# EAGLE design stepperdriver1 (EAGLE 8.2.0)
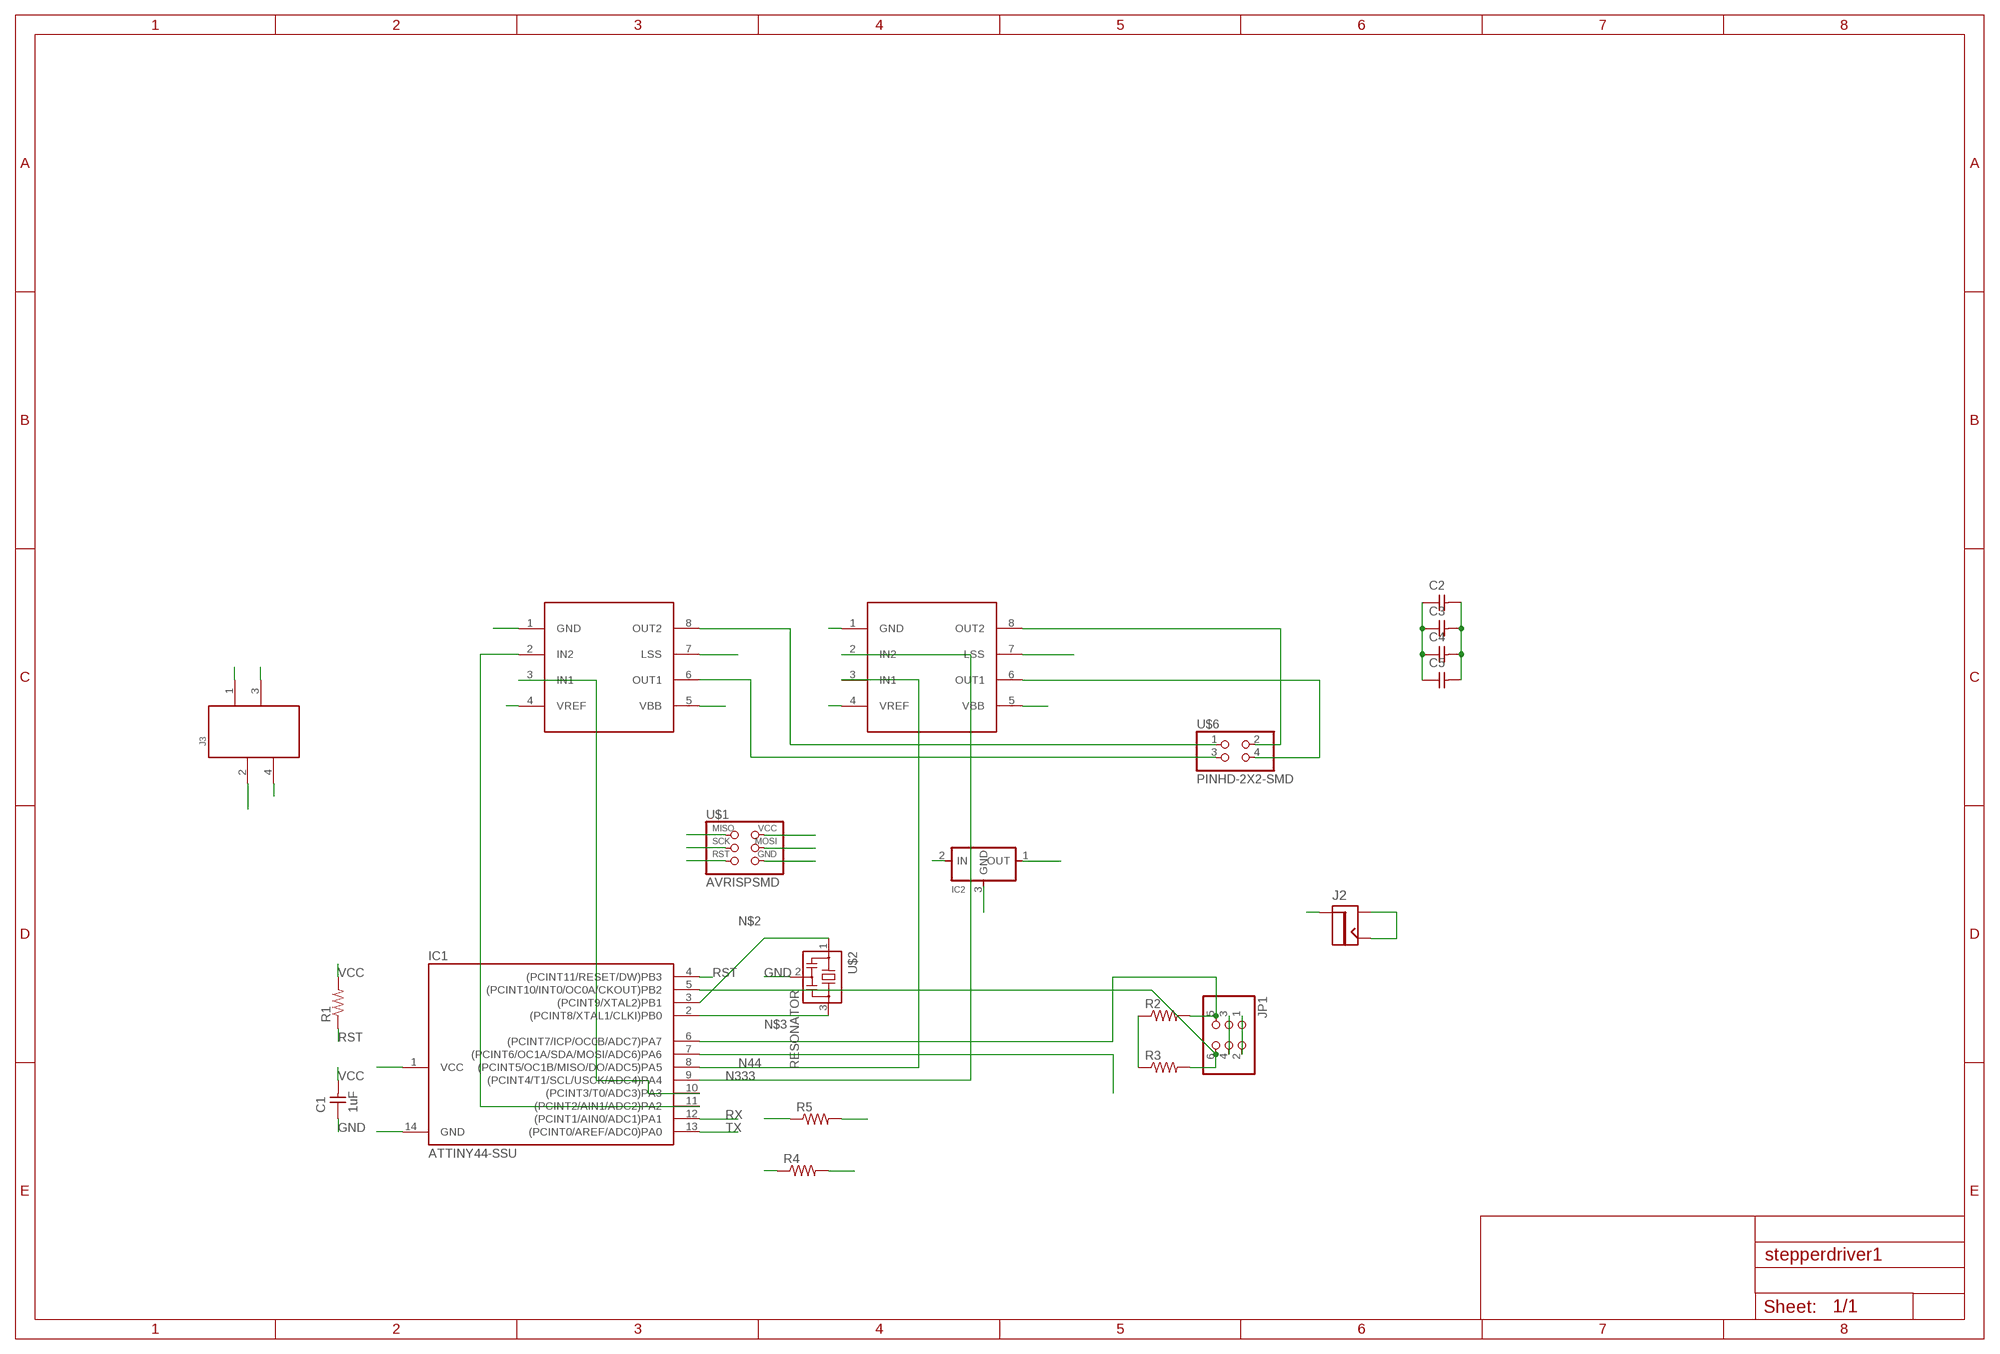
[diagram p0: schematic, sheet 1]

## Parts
C1  1uF  CAP-UNPOLARIZEDFAB  [C1206FAB]
C2  CAP-UNPOLARIZEDFAB  [C1206FAB]
C3  CAP-UNPOLARIZEDFAB  [C1206FAB]
C4  CAP-UNPOLARIZEDFAB  [C1206FAB]
C5  CAP-UNPOLARIZEDFAB  [C1206FAB]
IC1  ATTINY44-SSU  [SOIC14]
IC2  REGULATORSOT23  [SOT23]
J2  JACK2.1MM  [JACK_2.1MM]
J3  61000418321  [61000418321]
JP1  PINHD-2X3-SMD  [2X03SMD]
R1  RES-US1206FAB  [R1206FAB]
R2  RES-US1206FAB  [R1206FAB]
R3  RES-US1206FAB  [R1206FAB]
R4  RES-US1206FAB  [R1206FAB]
R5  RES-US1206FAB  [R1206FAB]
U$1  AVRISPSMD  [2X03SMD]
U$2  RESONATOR  [EFOBM]
U$4  A4953-H-BRIDGE-MOTOR-DRIVER  [SOIC8]
U$5  A4953-H-BRIDGE-MOTOR-DRIVER  [SOIC8]
U$6  PINHD-2X2-SMD  [2X02SMD]

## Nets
GND: C1.1 C2.1 C3.1 C4.1 C5.1 IC1.14(GND) IC2.3(GND) J2.CONTACT J2.SHUNT J3.2 JP1.1 JP1.2 R2.1 R3.1 R4.1 R4.2 R5.1 R5.2 U$1.6(GND) U$2.2 U$4.1(GND) U$4.7(LSS) U$5.1(GND) U$5.7(LSS)
MISO: IC1.8((PCINT5/OC1B/MISO/DO/ADC5)PA5) U$1.1(MISO) U$5.3(IN1)
MOSI: IC1.7((PCINT6/OC1A/SDA/MOSI/ADC6)PA6) U$1.4(MOSI)
N44: IC1.6((PCINT7/ICP/OC0B/ADC7)PA7) JP1.5 R2.2
N333: IC1.5((PCINT10/INT0/OC0A/CKOUT)PB2) JP1.6 R3.2
N$1: U$5.6(OUT1) U$6.4
N$2: IC1.3((PCINT9/XTAL2)PB1) U$2.1
N$3: IC1.2((PCINT8/XTAL1/CLKI)PB0) U$2.3
N$4: U$5.8(OUT2) U$6.2
N$5: U$4.8(OUT2) U$6.1
N$6: U$4.6(OUT1) U$6.3
N$9: IC1.10((PCINT3/T0/ADC3)PA3) U$4.3(IN1)
N$10: IC1.11((PCINT2/AIN1/ADC2)PA2) U$4.2(IN2)
RST: IC1.4((PCINT11/RESET/DW)PB3) R1.1 U$1.5(RST)
RX: IC1.12((PCINT1/AIN0/ADC1)PA1) J3.3
SCK: IC1.9((PCINT4/T1/SCL/USCK/ADC4)PA4) U$1.3(SCK) U$5.2(IN2)
TX: IC1.13((PCINT0/AREF/ADC0)PA0) J3.4
VBB: C2.2 C3.2 C4.2 C5.2 IC2.2(IN) J2.PIN U$4.5(VBB) U$5.5(VBB)
VCC: C1.2 IC1.1(VCC) IC2.1(OUT) J3.1 JP1.3 JP1.4 R1.2 U$1.2(VCC) U$4.4(VREF) U$5.4(VREF)

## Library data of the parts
C1-C5 = fab:CAP-UNPOLARIZED
IC1 = fab:ATTINY44
IC2 = fab:REGULATOR
J2 = fab:JACK
J3 = EAGLE-BOARD-TO-BOARD_CONNECTORS-rev16c:61000418321: WR-PHD 2.54mm SMT Pin Header, 4 Pins =>Code : Con_BTB_PHD_2.54_1_SMT_61000418321 Details see: http://katalog.we-online.de/en/em/610_0xx_182_21 Created 2014-05-29, Karrer Zheng 2014 (C) Würth Elektronik
JP1 = fab:PINHD-2X3-SMD: PIN HEADER
R1-R5 = fab:RES-US: Resistor (US Symbol)
U$1 = fab:AVRISP
U$2 = fab:RESONATOR
U$4 U$5 = fab:A4953-H-BRIDGE-MOTOR-DRIVER
U$6 = fab:PINHD-2X2-SMD

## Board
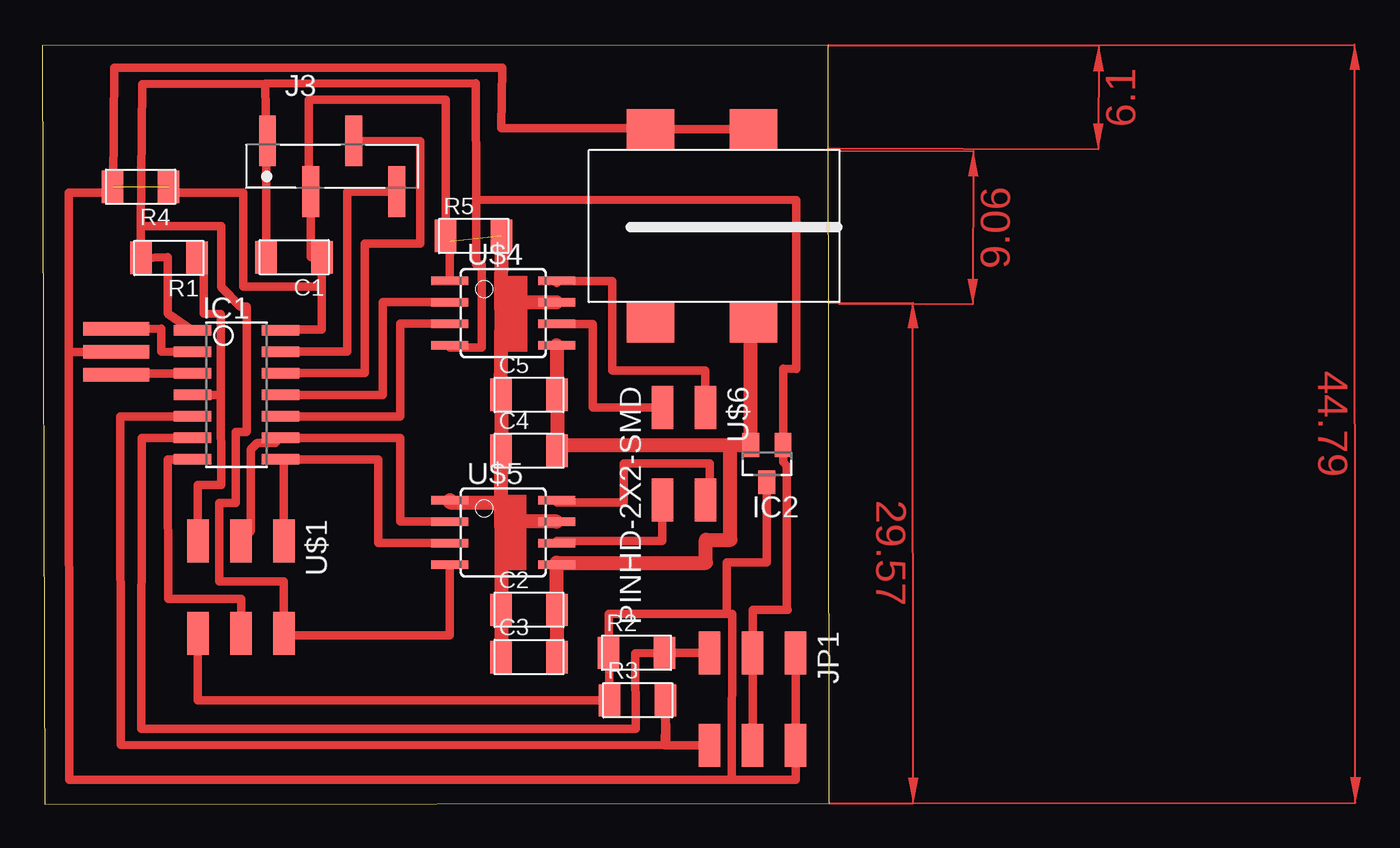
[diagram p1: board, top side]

Size 46.47 x 44.87 mm. Coordinates in mm from the lower left corner, seen from the top.
Outline: 0.14,0 46.47,0.08 46.42,44.87 0,44.84 0.14,0
Copper layers (1*16): Top 0.035mm / dielectric 1.5mm / Bottom 0.035mm
Design rules "default *": minimum track width 10mil, minimum drill 24mil, track to track 16mil, track to pad 16mil, pad to pad 16mil, via to via 16mil, smd to smd 16mil, copper to edge 40mil, drill to drill 8mil, minimum pad ring 10mil, minimum via ring 8mil, stop-mask expansion 4mil, vias tented up to drill 0mil, thermal gap 10mil

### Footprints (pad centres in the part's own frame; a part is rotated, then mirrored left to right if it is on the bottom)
C1206FAB = smd 1.27 x 1.905: 1 -1.651,0; 2 1.651,0
SOIC14 = smd 0.61 x 2.21: 1 -3.81,-2.603; 2 -2.54,-2.603; 3 -1.27,-2.603; 4 0,-2.603; 5 1.27,-2.603; 6 2.54,-2.603; 7 3.81,-2.603; 8 3.81,2.603; 9 2.54,2.603; 10 1.27,2.603; 11 0,2.603; 12 -1.27,2.603; 13 -2.54,2.603; 14 -3.81,2.603
SOT23 = smd 1 x 1.4: 1 -0.95,-1.1; 2 0.95,-1.1; 3 0,1.1
JACK_2.1MM = smd 2.388 x 2.794: CONTACT 5.766,-2.413; PIN -5.639,-2.413; PIN1 -5.639,3.683; SHUNT 5.766,3.683
61000418321 = smd 1 x 3: 1 -3.81,1.5; 2 -1.27,-1.5; 3 1.27,1.5; 4 3.81,-1.5
2X03SMD = smd 2.54 x 1.27: 1 -2.54,2.54; 2 2.92,2.54; 3 -2.54,0; 4 2.92,0; 5 -2.54,-2.54; 6 2.92,-2.54
R1206FAB = smd 1.27 x 1.905: 1 -1.651,0; 2 1.651,0
EFOBM = smd 0.8 x 3.9: 1 -1.35,0; 2 0,0; 3 1.35,0
SOIC8 = smd 0.5 x 2.2: 1 -1.905,-3.154; 2 -0.645,-3.154; 3 0.625,-3.154; 4 1.895,-3.154; 5 1.905,3.154; 6 0.635,3.154; 7 -0.635,3.154; 8 -1.905,3.154
2X02SMD = smd 2.54 x 1.27: 1 -2.54,1.27; 2 2.92,1.27; 3 -2.54,-1.27; 4 2.92,-1.27

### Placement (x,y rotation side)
C1  14.87,32.33 180 top
C2  28.74,11.51 0 top
C3  28.74,8.71 0 top
C4  28.74,20.9 0 top
C5  28.74,24.21 0 top
IC1  11.47,24.21 270 top
IC2  42.79,20.14 180 top
J2  39.59,34.12 90 top
J3  17.11,37.71 0 top
JP1  41.95,6.43 270 top
R1  7.47,32.3 180 top
R2  35.09,8.97 0 top
R3  35.15,6.16 0 top
R4  5.8,36.5 180 top
R5  25.47,33.59 0 top
U$1  11.72,13.03 270 top
U$2  4.36,26.75 90 top
U$4  27.22,29.03 270 top
U$5  27.22,16.08 270 top
U$6  37.88,20.9 270 top

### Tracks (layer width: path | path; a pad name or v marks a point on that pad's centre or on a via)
GND  (2 unrouted)
  Top 0.508: JP1.1 JP1.2 44.49,1.46 40.7,1.46 | IC2.3 42.79,14.3 40.42,14.3 40.42,11.25 | 40.42,11.25 33.44,11.25 R2.1 R3.1 9.17,6.15 U$1.6 | U$2.2 1.56,26.75 | 1.56,26.75 1.59,1.46 40.7,1.46 | 40.42,11.25 40.74,11.25 40.7,1.46 | 1.56,26.75 1.56,36.14 4.15,36.14 R4.2 4.18,36.5 4.24,43.52 27.17,43.52 27.1,39.95 35.9,39.95 J2.SHUNT J2.CONTACT | IC1.14 14.07,28.07 16.51,28.07 16.51,30.61 | 16.51,30.61 16.51,32.33 C1.1 15.84,32.33 J3.2 15.74,36.21 15.74,41.66 23.82,41.66 R5.1 24.06,33.25 U$4.1 | R4.1 7.46,36.14 11.85,36.14 11.85,30.61 16.51,30.61
  Top 0.813: 27.09,17.86 C4.1 C5.1 27.04,24.21 27.09,29.34 | 27.09,16.47 27.09,17.86 | 27.09,16.47 C2.1 C3.1 | U$5.1 24.06,17.86 27.09,17.86 | 27.09,29.34 R5.2 | U$4.7 27.41,29.67 27.09,29.34 | U$5.7 27.33,16.71 27.09,16.47
MISO
  Top 0.508: U$5.3 19.85,15.45 19.85,20.4 IC1.8 14.26,20.4 U$1.1
MOSI
  Top 0.508: IC1.7 7.4,20.4 7.44,12.15 11.76,12.15 U$1.4
N44
  Top 0.508: JP1.5 R2.2 35,8.93 35.03,4.47 5.86,4.47 5.88,21.67 IC1.6
N333
  Top 0.508: JP1.6 36.74,3.51 R3.2 36.84,3.51 4.62,3.52 4.61,22.94 IC1.5
N$1
  Top 0.508: U$5.6 30.37,15.57 36.61,15.57 U$6.4
N$2
  Top 0.508: U$2.1 3.85,25.48 IC1.3
N$3
  Top 0.508: IC1.2 7.02,26.77 7.02,28.12 U$2.3
N$4
  Top 0.508: U$5.8 30.37,17.86 34.33,17.86 34.33,20.14 39.41,20.14 39.41,17.6 39.15,17.6 U$6.2
N$5
  Top 0.508: 30.37,30.81 U$4.8 33.66,30.94 33.66,25.63 39.15,25.63 U$6.1
N$6
  Top 0.508: U$4.6 32.51,28.4 32.51,23.46 36.61,23.46 U$6.3
N$9
  Top 0.508: IC1.10 21.12,22.94 21.12,28.41 U$4.3
N$10
  Top 0.508: IC1.11 20.1,24.21 20.1,29.68 U$4.2
RST
  Top 0.508: U$1.5 9.18,18.87 10.55,18.87 10.53,24.2 | 10.53,24.2 IC1.4 | 10.53,24.2 10.54,28.98 9.54,29.02 9.54,32.3 R1.1
RX
  Top 0.508: J3.3 22.33,39.21 22.33,33.15 19.05,33.15 19.05,25.49 14.07,25.49 IC1.12
SCK
  Top 0.508: U$5.2 21.12,16.72 21.12,21.67 IC1.9 13.77,21.36 12.69,21.36 12.31,20.97 12.31,16.15 U$1.3
TX
  Top 0.508: J3.4 18,36.21 18,26.76 14.07,26.76 IC1.13
VBB
  Top 0.813: U$4.5 30.37,24.21 C5.2 C4.2 30.39,21.24 40.63,21.24 | C3.2 C2.2 30.37,11.51 U$5.5 30.37,14.29 39.18,14.29 39.18,15.65 40.63,15.65 40.63,21.24 | 40.63,21.24 IC2.2 41.84,28.49 J2.PIN
VCC
  Top 0.508: IC1.1 7.4,29.01 7.4,32.33 R1.2 5.82,34.18 | U$4.4 24.06,27 25.95,27 25.95,31.89 25.63,31.89 25.63,35.75 | U$5.4 24.06,9.98 14.26,9.98 U$1.2 14.26,13.18 10.45,13.2 10.45,17.83 11.43,17.83 11.43,22.01 12.04,22 12.07,22.03 12.07,29.43 11.69,29.43 10.55,30.57 10.55,34.18 5.82,34.18 | JP1.4 JP1.3 41.95,11.51 44.03,11.51 43.95,11.59 43.95,20.02 43.74,20.23 IC2.1 | 5.82,34.18 5.89,42.55 13.17,42.58 | 13.17,42.58 25.59,42.61 25.63,35.75 | IC2.1 43.54,21.24 | C1.2 13.22,39.13 J3.1 13.22,39.21 13.17,42.58 | IC2.1 43.74,25.77 44.53,25.73 44.53,35.71 25.63,35.75
(copper drawn outside any net)
  shapes: Top area x6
